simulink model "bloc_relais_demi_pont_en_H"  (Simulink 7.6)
settings: Solver=ode15s  StartTime=0.0  StopTime=1  RelTol=1e-3
libraries: fl_lib x14, nesl_utility x11, elec_lib x2, simulink x1

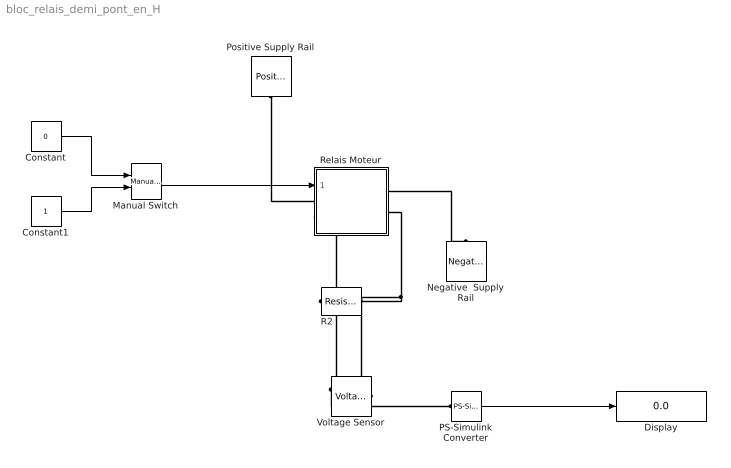
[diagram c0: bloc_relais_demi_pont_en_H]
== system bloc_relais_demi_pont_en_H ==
  Constant : Constant  Value=0
  Constant1 : Constant
  Display : Display
  Manual Switch : simulink/Signal Routing/Manual Switch  SystemSampleTime=-1  sw=1  action=0  varsize=off
  Negative  Supply Rail : elec_lib/Sources/Negative Supply Rail  DialogController=NetworkEngine.DynNeDlgSource  SystemSampleTime=-1  v0=-12 V  current_Log=off  voltage_Log=off  power_Log=off  LocalVarNames=|current|voltage|power  LocalVarDescs=|Current (A)|Voltage (V)|Power (W)  LocalVarLogging=[0 0 0]
  PS-Simulink Converter : nesl_utility/PS-Simulink Converter  DialogController=NetworkEngine.DynNeUtilDlgSource  SystemSampleTime=-1  PhysicalDomain=network_engine_domain  LeftPortType=input  RightPortType=output  SubClassName=ps_output  Unit=1  AffineConversion=off
  Positive Supply Rail : elec_lib/Sources/Positive Supply Rail  DialogController=NetworkEngine.DynNeDlgSource  SystemSampleTime=-1  v0=12 V  current_Log=off  voltage_Log=off  power_Log=off  LocalVarNames=|current|voltage|power  LocalVarDescs=|Current (A)|Voltage (V)|Power (W)  LocalVarLogging=[0 0 0]
  R2 : fl_lib/Electrical/Electrical Elements/Resistor  DialogController=NetworkEngine.DynNeDlgSource  SystemSampleTime=-1  R=10 kOhm  i_Log=off  v_Log=off  LocalVarNames=|i|v  LocalVarDescs=|i|v  LocalVarLogging=[0 0]
  Relais Moteur : Subsystem
  Voltage Sensor : fl_lib/Electrical/Electrical Sensors/Voltage Sensor  DialogController=NetworkEngine.DynNeDlgSource  SystemSampleTime=-1  i1_Log=off  v1_Log=off  LocalVarNames=|i1|v1  LocalVarDescs=|i1|v1  LocalVarLogging=[0 0]
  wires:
  PS-Simulink Converter/1 -> Display/1
  Constant1/1 -> Manual Switch/2
  Constant/1 -> Manual Switch/1
  Manual Switch/1 -> Relais Moteur/1(cde_sens)
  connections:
  R2/RConn1 -- Relais Moteur/LConn2 -- Voltage Sensor/LConn1
  Relais Moteur/RConn2 -- R2/LConn1 -- Voltage Sensor/RConn2
  Positive Supply Rail/RConn1 -- Relais Moteur/LConn1
  Relais Moteur/RConn1 -- Negative  Supply Rail/LConn1
  Voltage Sensor/RConn1 -- PS-Simulink Converter/LConn1

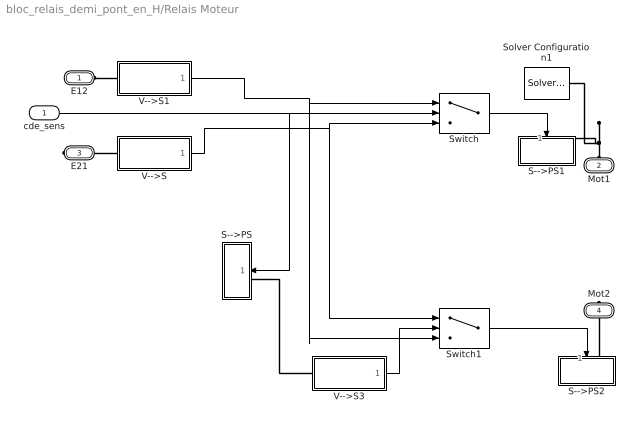
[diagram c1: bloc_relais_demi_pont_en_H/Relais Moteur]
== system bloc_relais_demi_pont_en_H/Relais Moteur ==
  cde_sens : Inport
  S-->PS : Subsystem
  S-->PS1 : Subsystem
  S-->PS2 : Subsystem
  Solver Configuration1 : nesl_utility/Solver Configuration  DialogController=NetworkEngine.DynNeUtilDlgSource  SystemSampleTime=-1  PhysicalDomain=network_engine_domain  LeftPortType=input  RightPortType=generic  SubClassName=solver  Accelerate=off  Profile=off  ResidualTolerance=1e-9  MaxNonlinIter=3  MaxModeIter=2  DoFixedCost=off  UseLocalSampling=off  DoDC=off  LinearAlgebra=Sparse  LocalSolverSampleTime=.001  LocalSolverChoice=NE_BACKWARD_EULER_ADVANCER  UseLocalSolver=off
  Switch : Switch  Threshold=0.5
  Switch1 : Switch  Threshold=0.5
  V-->S : Subsystem
  V-->S1 : Subsystem
  V-->S3 : Subsystem
  E12 : PMIOPort  Port=1  Side=Left
  Mot1 : PMIOPort  Port=2  Side=Left
  E21 : PMIOPort  Port=3  Side=Right
  Mot2 : PMIOPort  Port=4  Side=Right
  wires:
  V-->S/1(S) -> Switch/3, Switch1/1
  V-->S1/1(S) -> Switch/1, Switch1/3
  V-->S3/1(S) -> Switch1/2
  Switch/1 -> S-->PS1/1(S)
  cde_sens/1 -> Switch/2, S-->PS/1(S)
  Switch1/1 -> S-->PS2/1(S)
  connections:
  Mot1/RConn1 -- S-->PS1/LConn1 -- Solver Configuration1/RConn1
  S-->PS/LConn1 -- V-->S3/LConn1
  E12/RConn1 -- V-->S1/LConn1
  E21/RConn1 -- V-->S/LConn1
  Mot2/RConn1 -- S-->PS2/LConn1

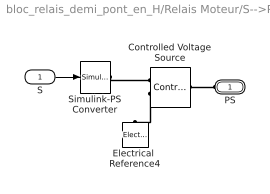
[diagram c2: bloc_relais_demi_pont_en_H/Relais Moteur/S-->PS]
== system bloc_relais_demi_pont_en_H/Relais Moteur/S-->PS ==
  S : Inport
  Controlled Voltage Source : fl_lib/Electrical/Electrical Sources/Controlled Voltage Source  DialogController=NetworkEngine.DynNeDlgSource  SystemSampleTime=-1  i_Log=off  v_Log=off  LocalVarNames=|i|v  LocalVarDescs=|i|v  LocalVarLogging=[0 0]
  Electrical  Reference4 : fl_lib/Electrical/Electrical Elements/Electrical Reference  DialogController=NetworkEngine.DynNeDlgSource  SystemSampleTime=-1  i_Log=off  LocalVarNames=|i  LocalVarDescs=|i  LocalVarLogging=0
  Simulink-PS Converter : nesl_utility/Simulink-PS Converter  DialogController=NetworkEngine.DynNeUtilDlgSource  SystemSampleTime=-1  PhysicalDomain=network_engine_domain  LeftPortType=input  RightPortType=output  SubClassName=ps_input  Unit=1  AffineConversion=off  InputFilterTimeConstant=.001  UdotUserProvided=0
  PS : PMIOPort  Port=1  Side=Left
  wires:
  S/1 -> Simulink-PS Converter/1
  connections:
  PS/RConn1 -- Controlled Voltage Source/LConn1
  Controlled Voltage Source/RConn2 -- Electrical  Reference4/LConn1
  Simulink-PS Converter/RConn1 -- Controlled Voltage Source/RConn1

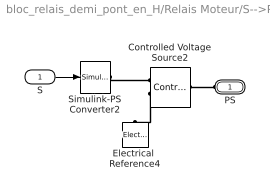
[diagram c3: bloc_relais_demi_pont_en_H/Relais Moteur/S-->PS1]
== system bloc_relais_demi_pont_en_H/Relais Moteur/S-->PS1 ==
  S : Inport
  Controlled Voltage Source2 : fl_lib/Electrical/Electrical Sources/Controlled Voltage Source  DialogController=NetworkEngine.DynNeDlgSource  SystemSampleTime=-1  i_Log=off  v_Log=off  LocalVarNames=|i|v  LocalVarDescs=|i|v  LocalVarLogging=[0 0]
  Electrical  Reference4 : fl_lib/Electrical/Electrical Elements/Electrical Reference  DialogController=NetworkEngine.DynNeDlgSource  SystemSampleTime=-1  i_Log=off  LocalVarNames=|i  LocalVarDescs=|i  LocalVarLogging=0
  Simulink-PS Converter2 : nesl_utility/Simulink-PS Converter  DialogController=NetworkEngine.DynNeUtilDlgSource  SystemSampleTime=-1  PhysicalDomain=network_engine_domain  LeftPortType=input  RightPortType=output  SubClassName=ps_input  Unit=1  AffineConversion=off  InputFilterTimeConstant=.001  UdotUserProvided=0
  PS : PMIOPort  Port=1  Side=Left
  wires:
  S/1 -> Simulink-PS Converter2/1
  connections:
  PS/RConn1 -- Controlled Voltage Source2/LConn1
  Controlled Voltage Source2/RConn2 -- Electrical  Reference4/LConn1
  Simulink-PS Converter2/RConn1 -- Controlled Voltage Source2/RConn1

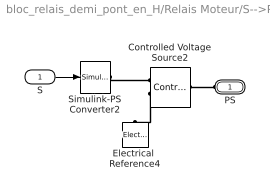
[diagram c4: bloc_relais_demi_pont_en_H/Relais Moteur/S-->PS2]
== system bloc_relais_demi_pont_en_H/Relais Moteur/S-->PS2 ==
  S : Inport
  Controlled Voltage Source2 : fl_lib/Electrical/Electrical Sources/Controlled Voltage Source  DialogController=NetworkEngine.DynNeDlgSource  SystemSampleTime=-1  i_Log=off  v_Log=off  LocalVarNames=|i|v  LocalVarDescs=|i|v  LocalVarLogging=[0 0]
  Electrical  Reference4 : fl_lib/Electrical/Electrical Elements/Electrical Reference  DialogController=NetworkEngine.DynNeDlgSource  SystemSampleTime=-1  i_Log=off  LocalVarNames=|i  LocalVarDescs=|i  LocalVarLogging=0
  Simulink-PS Converter2 : nesl_utility/Simulink-PS Converter  DialogController=NetworkEngine.DynNeUtilDlgSource  SystemSampleTime=-1  PhysicalDomain=network_engine_domain  LeftPortType=input  RightPortType=output  SubClassName=ps_input  Unit=1  AffineConversion=off  InputFilterTimeConstant=.001  UdotUserProvided=0
  PS : PMIOPort  Port=1  Side=Left
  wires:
  S/1 -> Simulink-PS Converter2/1
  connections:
  Simulink-PS Converter2/RConn1 -- Controlled Voltage Source2/RConn1
  Controlled Voltage Source2/RConn2 -- Electrical  Reference4/LConn1
  PS/RConn1 -- Controlled Voltage Source2/LConn1

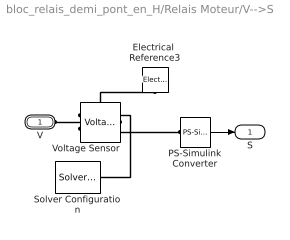
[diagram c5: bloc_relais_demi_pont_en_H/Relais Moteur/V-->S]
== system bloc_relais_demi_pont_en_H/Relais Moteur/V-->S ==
  Electrical  Reference3 : fl_lib/Electrical/Electrical Elements/Electrical Reference  DialogController=NetworkEngine.DynNeDlgSource  SystemSampleTime=-1  i_Log=off  LocalVarNames=|i  LocalVarDescs=|i  LocalVarLogging=0
  PS-Simulink Converter : nesl_utility/PS-Simulink Converter  DialogController=NetworkEngine.DynNeUtilDlgSource  SystemSampleTime=-1  PhysicalDomain=network_engine_domain  LeftPortType=input  RightPortType=output  SubClassName=ps_output  Unit=1  AffineConversion=off
  Solver Configuration : nesl_utility/Solver Configuration  DialogController=NetworkEngine.DynNeUtilDlgSource  SystemSampleTime=-1  PhysicalDomain=network_engine_domain  LeftPortType=input  RightPortType=generic  SubClassName=solver  Accelerate=off  Profile=off  ResidualTolerance=1e-9  MaxNonlinIter=3  MaxModeIter=2  DoFixedCost=off  UseLocalSampling=off  DoDC=off  LinearAlgebra=Sparse  LocalSolverSampleTime=.001  LocalSolverChoice=NE_BACKWARD_EULER_ADVANCER  UseLocalSolver=off
  Voltage Sensor : fl_lib/Electrical/Electrical Sensors/Voltage Sensor  DialogController=NetworkEngine.DynNeDlgSource  SystemSampleTime=-1  i1_Log=off  v1_Log=off  LocalVarNames=|i1|v1  LocalVarDescs=|i1|v1  LocalVarLogging=[0 0]
  V : PMIOPort  Port=1  Side=Left
  S : Outport
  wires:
  PS-Simulink Converter/1 -> S/1
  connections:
  Voltage Sensor/RConn2 -- Electrical  Reference3/LConn1
  Voltage Sensor/RConn1 -- PS-Simulink Converter/LConn1 -- Solver Configuration/RConn1
  V/RConn1 -- Voltage Sensor/LConn1

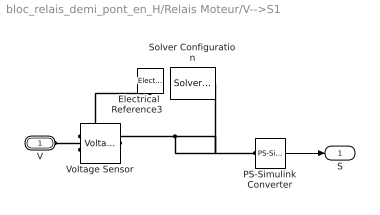
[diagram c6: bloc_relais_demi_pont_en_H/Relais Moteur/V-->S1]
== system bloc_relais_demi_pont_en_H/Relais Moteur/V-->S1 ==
  Electrical  Reference3 : fl_lib/Electrical/Electrical Elements/Electrical Reference  DialogController=NetworkEngine.DynNeDlgSource  SystemSampleTime=-1  i_Log=off  LocalVarNames=|i  LocalVarDescs=|i  LocalVarLogging=0
  PS-Simulink Converter : nesl_utility/PS-Simulink Converter  DialogController=NetworkEngine.DynNeUtilDlgSource  SystemSampleTime=-1  PhysicalDomain=network_engine_domain  LeftPortType=input  RightPortType=output  SubClassName=ps_output  Unit=1  AffineConversion=off
  Solver Configuration : nesl_utility/Solver Configuration  DialogController=NetworkEngine.DynNeUtilDlgSource  SystemSampleTime=-1  PhysicalDomain=network_engine_domain  LeftPortType=input  RightPortType=generic  SubClassName=solver  Accelerate=off  Profile=off  ResidualTolerance=1e-9  MaxNonlinIter=3  MaxModeIter=2  DoFixedCost=off  UseLocalSampling=off  DoDC=off  LinearAlgebra=Sparse  LocalSolverSampleTime=.001  LocalSolverChoice=NE_BACKWARD_EULER_ADVANCER  UseLocalSolver=off
  Voltage Sensor : fl_lib/Electrical/Electrical Sensors/Voltage Sensor  DialogController=NetworkEngine.DynNeDlgSource  SystemSampleTime=-1  i1_Log=off  v1_Log=off  LocalVarNames=|i1|v1  LocalVarDescs=|i1|v1  LocalVarLogging=[0 0]
  V : PMIOPort  Port=1  Side=Left
  S : Outport
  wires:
  PS-Simulink Converter/1 -> S/1
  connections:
  V/RConn1 -- Voltage Sensor/LConn1
  Voltage Sensor/RConn1 -- PS-Simulink Converter/LConn1 -- Solver Configuration/RConn1
  Voltage Sensor/RConn2 -- Electrical  Reference3/LConn1

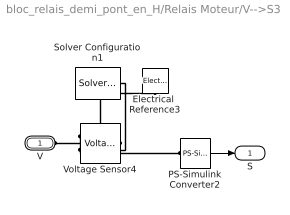
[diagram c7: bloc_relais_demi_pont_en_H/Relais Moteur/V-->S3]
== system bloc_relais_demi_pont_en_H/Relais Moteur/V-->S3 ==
  Electrical  Reference3 : fl_lib/Electrical/Electrical Elements/Electrical Reference  DialogController=NetworkEngine.DynNeDlgSource  SystemSampleTime=-1  i_Log=off  LocalVarNames=|i  LocalVarDescs=|i  LocalVarLogging=0
  PS-Simulink Converter2 : nesl_utility/PS-Simulink Converter  DialogController=NetworkEngine.DynNeUtilDlgSource  SystemSampleTime=-1  PhysicalDomain=network_engine_domain  LeftPortType=input  RightPortType=output  SubClassName=ps_output  Unit=1  AffineConversion=off
  Solver Configuration1 : nesl_utility/Solver Configuration  DialogController=NetworkEngine.DynNeUtilDlgSource  SystemSampleTime=-1  PhysicalDomain=network_engine_domain  LeftPortType=input  RightPortType=generic  SubClassName=solver  Accelerate=off  Profile=off  ResidualTolerance=1e-9  MaxNonlinIter=3  MaxModeIter=2  DoFixedCost=off  UseLocalSampling=off  DoDC=off  LinearAlgebra=Sparse  LocalSolverSampleTime=.001  LocalSolverChoice=NE_BACKWARD_EULER_ADVANCER  UseLocalSolver=off
  Voltage Sensor4 : fl_lib/Electrical/Electrical Sensors/Voltage Sensor  DialogController=NetworkEngine.DynNeDlgSource  SystemSampleTime=-1  i1_Log=off  v1_Log=off  LocalVarNames=|i1|v1  LocalVarDescs=|i1|v1  LocalVarLogging=[0 0]
  V : PMIOPort  Port=1  Side=Left
  S : Outport
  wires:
  PS-Simulink Converter2/1 -> S/1
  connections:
  Voltage Sensor4/RConn2 -- Electrical  Reference3/LConn1 -- Solver Configuration1/RConn1
  Voltage Sensor4/RConn1 -- PS-Simulink Converter2/LConn1
  V/RConn1 -- Voltage Sensor4/LConn1
